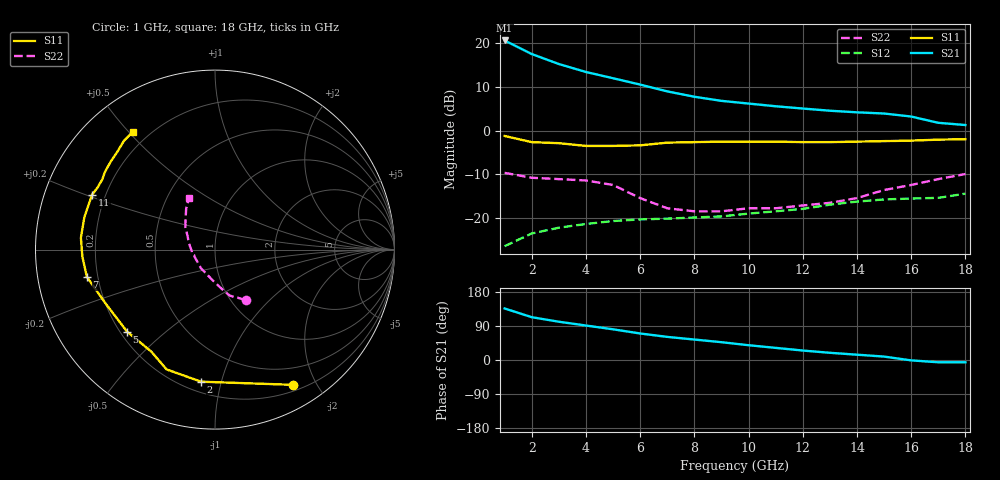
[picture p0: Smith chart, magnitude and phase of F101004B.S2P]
!ATF-10100
!S-PARAMETERS at Vds=4V  Id=70mA.  LAST UPDATED 07-22-92
# ghz s ma r 50
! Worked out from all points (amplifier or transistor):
!   18 points, 1 GHz to 18 GHz, reference 50 ohm
!   highest |S21| = 20.6 dB at 1 GHz (marker M1)
!   |S21| within 3 dB of that: start of sweep to 1.967 GHz
!   unconditionally stable (mu >= 1): 8.547 GHz to 13.8 GHz; 16.51 GHz to end of sweep
!   at 4 GHz: K = 0.69, MSG = 17.4 dB, |S12| = -21.3 dB
!   at 10 GHz: K = 1.02, MAG = 11.7 dB, |S12| = -18.9 dB
!   at 18 GHz: K = 1.00, MAG = 7.4 dB, |S12| = -14.4 dB
!   S11 on the Smith chart (normalised r, x): 1 GHz: 0.27, -1.70; 2 GHz: 0.27, -0.86; 5 GHz: 0.23, -0.38; 7 GHz: 0.16, -0.10; 11 GHz: 0.15, +0.21; 18 GHz: 0.14, +0.51
1  0.87 -60.0  10.72 136.0  0.048 55.0  0.33 -59.0
2  0.74 -96.0  7.5 113.0  0.067 43.0  0.29 -66.0
3  0.72 -112.0  5.77 101.0  0.078 39.0  0.28 -69.0
4  0.67 -122.0  4.68 91.0  0.086 38.0  0.27 -72.0
5  0.67 -137.0  3.97 81.0  0.093 36.0  0.24 -77.0
6  0.68 -154.0  3.36 70.0  0.097 35.0  0.17 -95.0
7  0.73 -168.0  2.81 61.0  0.099 33.0  0.13 -127.0
8  0.74 -177.0  2.44 54.0  0.102 31.0  0.12 -159.0
9  0.75 175.0  2.19 47.0  0.105 31.0  0.12 -165.0
10  0.75 166.0  2.04 39.0  0.113 29.0  0.13 -171.0
11  0.75 156.0  1.9 32.0  0.12 27.0  0.13 -177.0
12  0.74 152.0  1.79 25.0  0.128 26.0  0.14 173.0
13  0.74 148.0  1.69 19.0  0.143 25.0  0.15 166.0
14  0.75 145.0  1.62 14.0  0.155 24.0  0.17 154.0
15  0.76 140.0  1.57 9.0  0.164 21.0  0.21 142.0
16  0.77 135.0  1.45 -1.0  0.168 18.0  0.24 133.0
17  0.79 130.0  1.23 -6.0  0.171 18.0  0.28 125.0
18  0.8 125.0  1.16 -6.0  0.191 18.0  0.32 117.0
